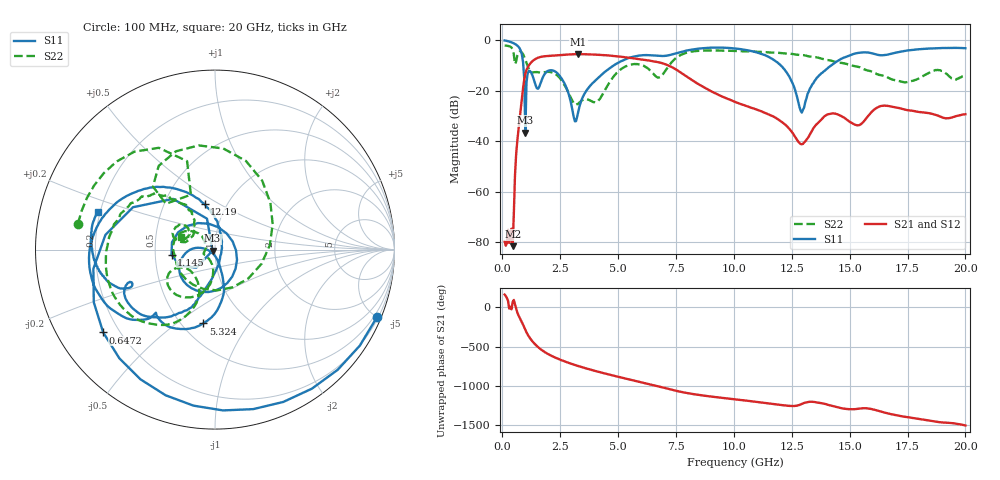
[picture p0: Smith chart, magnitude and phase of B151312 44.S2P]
!  2-Port S-parameters saved by WinCal
! VAR MeasName=S-Parameters (CALIBRATED_DATA) read from VNA (N5244A)
! VAR MeasDate=12/8/2015 5:47:21 PM
! VAR NAME=B151312 44
! VAR FILENAME=B151312 44.S2P
! VAR DATE=12/8/2015 5:47:21 PM
! VAR PHYS_PORTS=1,2
# Hz S DB R 50
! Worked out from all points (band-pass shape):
!   401 points, 100 MHz to 20 GHz, reference 50 ohm
!   highest |S21| = -5.63 dB at 3.284 GHz (marker M1); lowest = -81.6 dB at 448.2 MHz (marker M2)
!   |S21| within 3 dB of the highest: 1.276 GHz to 6.636 GHz (5.36 GHz wide, 135 % of centre)
!   lowest |S11| = -36.6 dB at 995.5 MHz (marker M3), VSWR 1.03, Z = 48.7 - j0.596 ohm
!   |S11| at or under -10 dB: 906.2 MHz to 4.823 GHz (3.917 GHz wide, 137 % of centre); 12.02 GHz to 14.21 GHz (2.194 GHz wide, 16.7 % of centre)
!   |S22| runs from -25.7 to -2.2 dB; largest |S21 - S12| = 0.0018
!   S11 on the Smith chart (normalised r, x): 100 MHz: 0.29, -4.99; 647.2 MHz: 0.14, -0.32; 1.145 GHz: 0.61, -0.04; 5.324 GHz: 0.63, -0.63; 12.19 GHz: 0.79, +0.43; 20 GHz: 0.19, +0.15
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1e8  -0.20 -22.6  -79.58 163.9  -79.08 165.5  -2.19 169.3
4.4825e8  -1.13 -97.9  -81.57 69.3  -86.30 55.0  -3.77 118.9
6.4725e8  -2.21 -143.5  -39.98 -62.5  -39.90 -62.3  -6.14 134.5
8.4625e8  -5.78 152.7  -23.08 171.4  -23.08 171.4  -4.96 85.3
9.955e8  -36.62 -155.5  -13.43 73.0  -13.43 73.0  -7.87 40.2
1.14475e9  -12.26 -173.5  -10.09 -10.2  -10.09 -10.3  -11.34 -17.0
1.3935e9  -16.55 103.8  -7.75 -103.7  -7.75 -103.7  -12.74 -122.2
1.74175e9  -14.97 -57.5  -6.55 168.1  -6.55 168.1  -12.86 -170.9
2.33875e9  -12.84 -150.9  -6.11 72.8  -6.11 72.8  -13.75 151.6
3.284e9  -28.30 -86.3  -5.63 -28.5  -5.63 -28.5  -25.23 -175.8
3.43325e9  -23.49 -75.5  -5.64 -42.1  -5.64 -42.1  -23.92 -166.3
4.22925e9  -14.26 -75.9  -5.89 -107.8  -5.89 -107.8  -23.14 -110.6
5.32375e9  -7.61 -99.0  -6.87 171.9  -6.84 171.8  -10.46 -117.4
6.7665e9  -6.28 -132.6  -8.86 71.6  -8.85 71.5  -14.87 -133.7
7.81125e9  -4.51 -138.9  -13.54 -3.2  -13.51 -3.5  -5.52 -127.8
1.005e10  -3.37 171.9  -24.49 -93.4  -24.48 -93.6  -4.33 -178.4
1.218925e10  -11.68 102.9  -33.24 -170.6  -33.28 -170.5  -5.34 154.0
1.29355e10  -28.73 -8.2  -41.26 -150.9  -41.31 -150.4  -5.94 144.1
1.338325e10  -17.65 -91.0  -35.79 -123.8  -35.73 -123.8  -6.69 138.3
1.4826e10  -6.73 -125.3  -31.15 145.5  -31.06 145.7  -9.41 127.7
1.67165e10  -5.67 -156.0  -26.21 82.8  -26.11 82.1  -15.13 130.5
2e10  -3.26 162.3  -29.37 -66.1  -29.47 -66.6  -13.83 159.6
